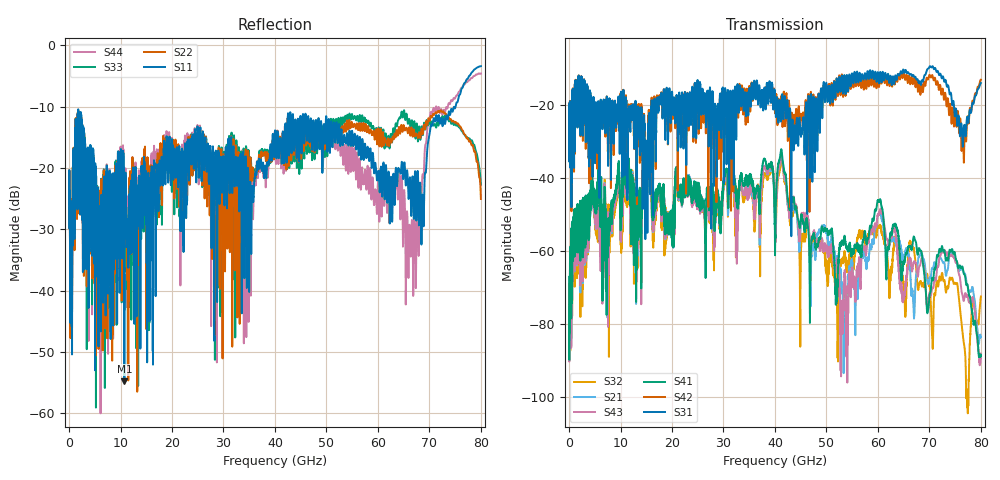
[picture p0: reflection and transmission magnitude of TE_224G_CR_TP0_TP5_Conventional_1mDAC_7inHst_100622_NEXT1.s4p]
!! Reference: tracy_3df_01_2211
!! CHANNEL DESCRIPTION: TP0_TP5 CR Channel using 1meter DAC, Conventional 7.6dB Host
!! MODEL DESCRIPTION: s4p, NEXT1
!! CONNECTOR DESCRIPTION: OSFP 200G SMT
!! CABLE DESCRIPTION: 1meter 26AWG Cable
!! MODEL STATUS: Developmental
!! PORT DEFINITIONS:
!! Port  1  ----->  Side A  Side B  <-----  Port  2
!! Port  3  ----->  Side A  Side B  <-----  Port  4
# Hz S MA R 50
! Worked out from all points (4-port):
!   8000 points, 10 MHz to 80 GHz, reference 50 ohm
!   strongest paths, dB at 10 MHz, 20.01 GHz, 40.01 GHz, 60.01 GHz, 80 GHz:
!     S31: -26.6, -16.2, -17.4, -11.0, -13.9
!     S42: -26.6, -16.9, -22.1, -12.9, -12.9
!     S41: -84.4, -56.0, -61.1, -46.0, -88.6
!     S43: -86.2, -55.6, -51.5, -49.9, -88.1
!     S21: -86.2, -56.1, -52.4, -50.0, -83.5
!     S32: -87.7, -55.5, -50.4, -53.5, -72.4
!   lowest |S11| = -54.8 dB at 10.74 GHz (marker M1), VSWR 1.00, Z = 50.2 + j0.0965 ohm
!   |S11| at or under -10 dB: start of sweep to 75.09 GHz
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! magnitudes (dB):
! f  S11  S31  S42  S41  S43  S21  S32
! 10 MHz  -24.3  -26.6  -26.6  -84.4  -86.2  -86.2  -87.7
! 10.74 GHz  -54.8  -25.2  -27.4  -35.5  -37.8  -37.4  -39.6
! 41.21 GHz  -17.2  -23.2  -17.7  -32.0  -33.3  -33.4  -34.9
! 52.94 GHz  -13.8  -12.1  -11.9  -57.4  -82.8  -68.6  -62.2
! 60.28 GHz  -22.9  -13.3  -14.2  -46.2  -49.2  -49.6  -53.4
! 67.12 GHz  -22.2  -12.3  -12.9  -56.5  -62.9  -75.9  -61.0
! 80 GHz  -3.4  -13.9  -12.9  -88.6  -88.1  -83.5  -72.4
